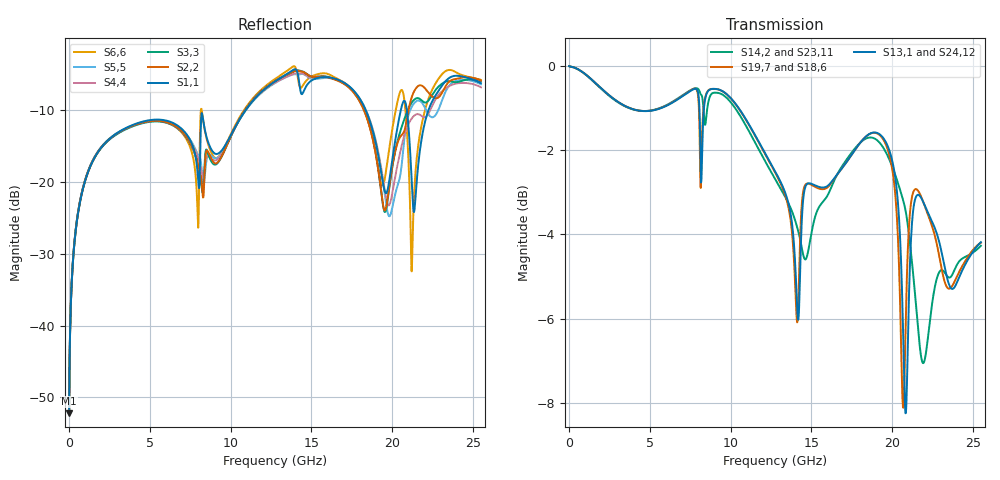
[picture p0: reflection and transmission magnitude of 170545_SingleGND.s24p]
!  COPYRIGHT 2014, BY MOLEX INCORPORATED
!  ALL INTERNATIONAL RIGHTS RESERVED
!  THIS FILE CONTAINS MOLEX INCORPORATED CONFIDENTIAL INFORMATION
! >>>>>>>>>>>>>>>>  USER AGREEMENT  <<<<<<<<<<<<<<<<<<<
! The information on this disk is the property of MOLEX Incorporated
! and  has been provided to you free of charge. Molex does not
! guarantee that the information is error-free, nor does MOLEX  make
! any representations, warranty or guarantee that the information is
! accurate, correct, reliable or up-to-date. MOLEX expressly
! disclaims all implied warranties regarding this information,
! including but not limited to any implied  warranties of
! merchantability or fitness for a particular purpose. MOLEX does
! not warrant that this file will work correctly in your multi- user
! or network environment.
! Touchstone file from project: 170545_SingleGND
! Exported from HFSS 2014
! MODEL TYPE: S-parameter
! MODEL FORMAT: Touchstone (*.sNp)
! MODEL BASIS: Analytical 3-D field solution
! BANDWIDTH: DC  25.48 GHz
! RESOLUTION: 10 MHz steps
! REFERENCE: 50 ohms
! NUMBER OF CHANNELS: 6 differential
! NUMBER OF PORTS: 24 single-ended
! CHANNEL TYPE: Coupled pairs + reference
! VALIDATION: NA
! MODEL APPLICATION: Vertical (nominal)
! This model has been verified as passive by HFSS's passivity checker.
! MODEL DESCRIPTION:
! This models consists of six differential channels.  Differential channels 1, 2 and 3 are
! positioned along one side of the connector while channels 4, 5 and 6 are positioned along
! the opposite side.  The six channels together are physically arranged in a 3x2 layout
! within the connector footprint and lead frame.  In addition to the connector geometry,
! a portion of the edge card was solved with the connector model.
! Further information regarding this connector series and other
! related Molex connectors can be found at http://www.molex.com/.
! Molex Part Numbers: 76693, 170545, 170682, 171852
! IMPORTANT NOTE: This model should not be used to evaluate
! electrical signals with greater than 25 GHz of frequency content.
! MODEL SKETCH
! < For best results, view these charts in a simple text
! editor such as notepad.  Text editors that automatically adjust spacing will
! make the columns mis-align. >
!  |  Edge card  |
!  Host board-side
!  terminals
! CONNECTION SKETCH
! < For best results, view these charts in a simple text
! editor such as notepad.  Text editors that automatically adjust spacing will
! make the columns mis-align. >
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# GHZ S MA R 50.000000
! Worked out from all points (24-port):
!   1274 points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, 20 MHz to 25.48 GHz, reference 50 ohm
!   strongest paths, dB at 20 MHz, 6.38 GHz, 12.76 GHz, 19.12 GHz, 25.48 GHz:
!     S13,1: 0.0, -0.9, -2.5, -1.6, -4.2
!     S19,7: 0.0, -0.9, -2.5, -1.6, -4.2
!     S24,12: 0.0, -0.9, -2.5, -1.7, -4.2
!     S18,6: 0.0, -0.8, -2.6, -1.7, -4.2
!     S14,2: 0.0, -0.9, -2.7, -1.8, -4.3
!     S23,11: 0.0, -0.9, -2.6, -1.8, -4.5
!   lowest |S11| = -52.2 dB at 20 MHz (marker M1), VSWR 1.00, Z = 50 + j0.244 ohm
!   |S11| at or under -10 dB: start of sweep to 10.95 GHz; 18.35 GHz to 20.53 GHz (2.181 GHz wide, 11.2 % of centre); 20.9 GHz to 22.25 GHz (1.345 GHz wide, 6.24 % of centre)
